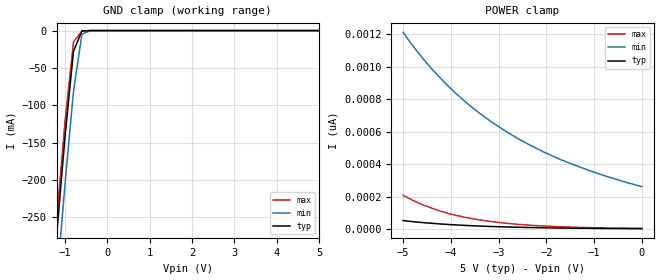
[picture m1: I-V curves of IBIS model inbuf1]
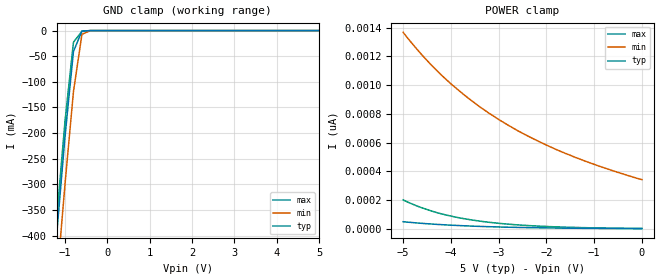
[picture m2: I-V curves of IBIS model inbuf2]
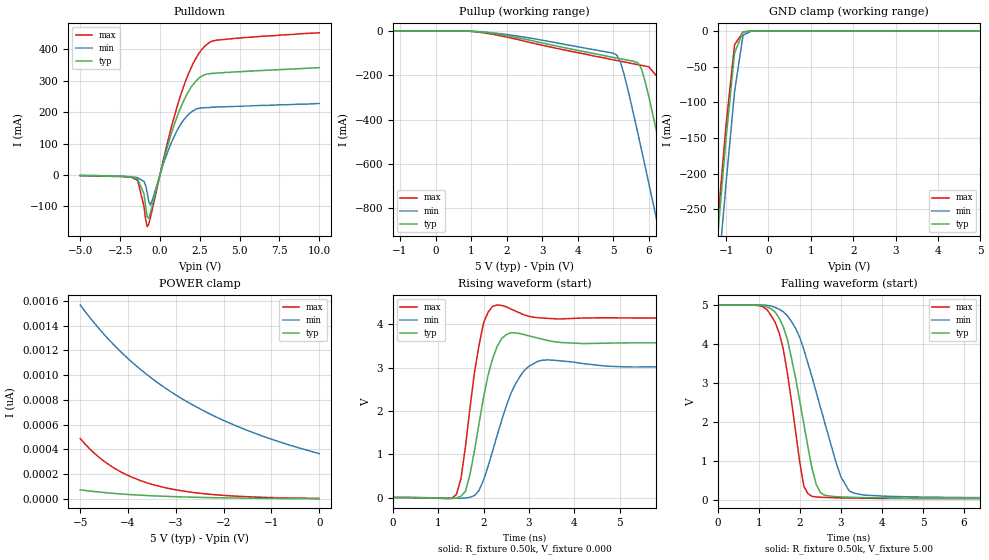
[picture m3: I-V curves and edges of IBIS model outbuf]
| IBIS file 61244l.ibs created by s2ibis2 version 1.0
| North Carolina State University Electronics Research Laboratory  1995
[IBIS ver]   2.1
[File name]   74fct16244t.ibs
[File Rev]   0.1
[Date]   Wednesday, April 16, 1997
[Source]   IDT
[Notes]   1. Temp typ=25C, min=100C, max=0C 2. Ramp rates based on 500
   ohm load
[Copyright]   Copyright 1997, Integrated Device Technology, Inc.
[Disclaimer] Integrated Device Technology, Inc. ("IDT") hereby grants the
   user of this IBIS model a non-exclusive, nontransferable
   license to use this IBIS model under the following terms.
   The user is granted this license only to use the IBIS model
   and is not granted rights to sell, copy (except as needed to
   run the IBIS model), rent, lease or sub-license the IBIS model
   in whole or in part, or in modified form to anyone.
   The User may modify the IBIS model to suit its specific
   applications, but rights to derivative works and such
   modifications shall belong to IDT.
   This IBIS model is provided on an "AS IS" basis and IDT
   makes absolutely no warranty with respect to the information
   contained herein. IDT DISCLAIMS AND CUSTOMER WAIVES ALL
   WARRANTIES, EXPRESS AND IMPLIED, INCLUDING WARRANTIES OF
   MERCHANTABILITY AND FITNESS FOR A PARTICULAR PURPOSE. THE
   ENTIRE RISK AS TO QUALITY AND PERFORMANCE IS WITH THE
   USER ACCORDINGLY, IN NO EVENT SHALL IDT BE LIABLE
   FOR ANY DIRECT OR INDIRECT DAMAGES, WHETHER IN CONTRACT OR
   TORT, INCLUDING ANY LOST PROFITS OR OTHER INCIDENTAL,
   CONSEQUENTIAL, EXEMPLARY, OR PUNITIVE DAMAGES ARISING OUT OF
   THE USE OR APPLICATION OF THE IBIS model.  Further, IDT
   reserves the right to make changes without notice to any
   product herein to improve reliability, function, or design.
   IDT does not convey any license under patent rights or
   any other intellectual property rights, including those of
   third parties. IDT is not obligated to provide maintenance
   or support for the licensed IBIS model.
|   Component IDT54/74FCT16244T/AT/CT/ET
[Component]   IDT54/74FCT16244T/AT/CT/ET
[Manufacturer]   Integrated Device Technology Inc.
[Package]
| Following package parameters are for SO48-2(TSSOP) package
|[Package]
|| variable   typ   min   max
|R_pkg   15.00m   10.00m   20.00m
|L_pkg   2.30nh   1.40nh   4.50nH
|C_pkg   0.40pF   0.35pF   0.60pF
| Following package parameters are for SO48-1(SSOP), E48-1(CERPAK) packages
| variable   typ   min   max
R_pkg   15.00m   10.00m   20.00m
L_pkg   2.90nH   1.50nH   5.60nH
C_pkg   0.40pF   0.26pF   0.50pF
[Pin]  signal_name   model_name   R_pin   L_pin   C_pin
1   1OEB   inbuf1
2   1Y1   outbuf
3   1Y2   outbuf
4   GND   GND
5   1Y3   outbuf
6   1Y4   outbuf
7   VCC   POWER
8   2Y1   outbuf
9   2Y2   outbuf
10   GND   GND
11   2Y3   outbuf
12   2Y4   outbuf
13   3Y1   outbuf
14   3Y2   outbuf
15   GND   GND
16   3Y3   outbuf
17   3Y4   outbuf
18   VCC   POWER
19   4Y1   outbuf
20   4Y2   outbuf
21   GND   GND
22   4Y3   outbuf
23   4Y4   outbuf
24   4OEB   inbuf1
25   3OEB   inbuf1
26   4A4   inbuf2
27   4A3   inbuf2
28   GND   GND
29   4A2   inbuf2
30   4A1   inbuf2
31   VCC   POWER
32   3A4   inbuf2
33   3A3   inbuf2
34   GND   GND
35   3A2   inbuf2
36   3A1   inbuf2
37   2A4   inbuf2
38   2A3   inbuf2
39   GND   GND
40   2A2   inbuf2
41   2A1   inbuf2
42   VCC   POWER
43   1A4   inbuf2
44   1A3   inbuf2
45   GND   GND
46   1A2   inbuf2
47   1A1   inbuf2
48   2OEB   inbuf1
| Models and submodels in the file (3): inbuf1 (Input), inbuf2 (Input), outbuf (3-state)
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| in   IN1   dummy_model
| oe   OE1   dummy_model
|   Model inbuf1
[Model]   inbuf1
Model_type   Input
Vinl =  0.800V
Vinh =  2.000V
C_comp   3.00pF   NA   NA
[Temperature Range]   25.00   100.00   0.000
[Voltage Range]   5.00V   4.50V   5.50V
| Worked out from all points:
|   GND clamp passes 1 mA (typ) near -0.60 V on its own axis
[GND_clamp]
| voltage   I(typ)   I(min)   I(max)
-5V       -3.018A    -3.076A    -2.999A
-1.4V     -415mA     -480mA     -394mA
-1.2V     -276mA     -341mA     -255mA
-1V       -142mA     -206mA     -122mA
-800mV    -27.87mA   -81.82mA   -15.26mA
-600mV    -480uA     -4.848mA   -551uA
-400mV    -1.016uA   -20.86uA   -873nA
5V        1.855pA    303pA      2.085pA
[POWER_clamp]
| voltage   I(typ)   I(min)   I(max)
-5V       51.46pA    1.212nA    208pA
-4.6V     39.61pA    1.056nA    150pA
-4.4V     34.75pA    987pA      128pA
-4.1V     28.53pA    894pA      99.73pA
-3.9V     25.02pA    837pA      84.6pA
-3.6V     20.53pA    760pA      66.05pA
-3.1V     14.75pA    650pA      43.65pA
-2.8V     12.09pA    593pA      34.01pA
-2.4V     9.265pA    526pA      24.35pA
-1.7V     5.808pA    428pA      13.54pA
-800mV    3.178pA    330pA      6.324pA
0V        1.855pA    261pA      3.199pA
|   Model inbuf2
[Model]   inbuf2
Model_type   Input
Vinl =  0.800V
Vinh =  2.000V
C_comp   3.00pF   NA   NA
[Temperature Range]   25.00   100.00   0.000
[Voltage Range]   5.00V   4.50V   5.50V
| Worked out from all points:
|   GND clamp passes 1 mA (typ) near -0.60 V on its own axis
[GND_clamp]
| voltage   I(typ)   I(min)   I(max)
-5V       -4.387A    -4.471A    -4.36A
-1.4V     -604mA     -698mA     -573mA
-1.2V     -402mA     -496mA     -371mA
-1V       -207mA     -300mA     -177mA
-800mV    -40.8mA    -119mA     -22.8mA
-600mV    -973uA     -7.222mA   -1.303mA
-400mV    -6.41uA    -46.07uA   -11.93uA
5V        1.965pA    393pA      2.176pA
[POWER_clamp]
| voltage   I(typ)   I(min)   I(max)
-5V       50.2pA     1.366nA    202pA
-4.6V     38.73pA    1.207nA    146pA
-4.4V     34.01pA    1.136nA    124pA
-4.1V     27.98pA    1.039nA    97.02pA
-3.6V     20.21pA    900pA      64.36pA
-3.4V     17.74pA    850pA      54.59pA
-3V       13.67pA    761pA      39.26pA
-2.6V     10.54pA    683pA      28.2pA
-2.3V     8.67pA     631pA      22pA
-1.6V     5.503pA    525pA      12.31pA
-900mV    3.5pA      437pA      6.893pA
0V        1.965pA    343pA      3.278pA
|   Model outbuf
[Model]   outbuf
Model_type   3-state
Polarity   Non-Inverting
Enable   Active-High
Vinl =  0.800V
Vinh =  2.000V
C_comp   3.00pF   NA   NA
[Temperature Range]   25.00   100.00   0.000
[Voltage Range]   5.00V   4.50V   5.50V
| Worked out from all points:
|   slope of the pulldown table from 0 to 0.75 V, typ, clamps not added: 5.47 ohm
|   slope of the pullup table from 0 to 0.75 V, typ, clamps not added: 13.5 kohm
|   GND clamp passes 1 mA (typ) near -0.59 V on its own axis
|   rising waveform, R_fixture 0.50k, V_fixture 0.000: 20-80 % time 375ps typ, 548ps min, 314ps max; typ from 0 V to 3.57 V
|   falling waveform, R_fixture 0.50k, V_fixture 5.00: 20-80 % time 538ps typ, 813ps min, 427ps max; typ from 5 V to 0.048 V
[Pulldown]
| voltage   I(typ)   I(min)   I(max)
-5V       -1mA       -1mA       -2mA
-1.4V     -12.2mA    -8mA       -16.2mA
-1V       -60mA      -20.5mA    -100mA
-800mV    -133mA     -55.02mA   -164mA
-700mV    -138mA     -84.63mA   -156mA
-600mV    -121mA     -94.98mA   -136mA
400mV     77.42mA    61.63mA    88.42mA
1.2V      202mA      153mA      238mA
2.1V      289mA      205mA      357mA
2.8V      320mA      215mA      410mA
3.6V      325mA      217mA      430mA
10V       342mA      228mA      453mA
[Pullup]
| voltage   I(typ)   I(min)   I(max)
-5V       -22.81pA   -213pA     -284pA
1V        -1.033mA   -848uA     -1.818mA
5V        -119mA     -100mA     -130mA
5.2V      -125mA     -138mA     -136mA
5.3V      -128mA     -191mA     -139mA
5.8V      -172mA     -538mA     -155mA
6V        -294mA     -685mA     -161mA
6.4V      -582mA     -982mA     -236mA
6.8V      -881mA     -1.285A    -514mA
7.2V      -1.183A    -1.591A    -812mA
7.6V      -1.487A    -1.898A    -1.114A
10V       -3.347A    -3.753A    -2.965A
[GND_clamp]
| voltage   I(typ)   I(min)   I(max)
-5V       -3.225A    -3.259A    -3.225A
-1.4V     -433mA     -494mA     -416mA
-1.2V     -289mA     -351mA     -270mA
-1V       -150mA     -213mA     -131mA
-800mV    -30.94mA   -85.08mA   -19.24mA
-600mV    -1.072mA   -5.816mA   -1.489mA
-400mV    -7.978uA   -50.35uA   -16.99uA
5V        2.361pA    421pA      2.955pA
[POWER_clamp]
| voltage   I(typ)   I(min)   I(max)
-5V       73.75pA    1.567nA    488pA
-4.8V     64.14pA    1.465nA    404pA
-4.6V     55.79pA    1.372nA    334pA
-4.4V     48.53pA    1.286nA    277pA
-4.1V     39.37pA    1.169nA    208pA
-3.6V     27.8pA     1.003nA    130pA
-3.4V     24.19pA    944pA      108pA
-3V       18.32pA    840pA      74.07pA
-2.3V     11.29pA    689pA      38.46pA
-1.7V     7.474pA    584pA      21.99pA
-900mV    4.33pA     470pA      10.5pA
0V        2.361pA    366pA      4.626pA
[Ramp]
| variable   typ   min   max
dV/dt_r   2.14/0.38n   1.81/0.55n   2.49/0.31n
dV/dt_f   2.97/0.54n   2.67/0.77n   3.27/0.44n
R_load = 0.50k
[Rising Waveform]
R_fixture = 0.50k
V_fixture = 0.000
| time   V(typ)   V(min)   V(max)
0s        0V         0V         0V
1.4ns     -14.81mV   -17.58mV   72.21mV
1.6ns     143mV      -14.15mV   1.18V
1.9ns     1.712V     165mV      3.518V
2ns       2.319V     405mV      4.035V
2.2ns     3.209V     1.076V     4.415V
2.4ns     3.672V     1.785V     4.434V
2.7ns     3.801V     2.616V     4.305V
3.2ns     3.68V      3.146V     4.151V
9.9ns     3.57V      3.022V     4.145V
[Falling Waveform]
R_fixture = 0.50k
V_fixture = 5.00
| time   V(typ)   V(min)   V(max)
0s        5V         5V         5V
1.1ns     4.986V     4.995V     4.954V
1.4ns     4.817V     4.937V     4.556V
1.7ns     4.114V     4.724V     3.248V
2.1ns     1.954V     3.857V     361mV
2.3ns     817mV      3.153V     101mV
2.5ns     203mV      2.395V     80.66mV
3ns       89.02mV    607mV      61.7mV
3.3ns     77.02mV    192mV      56.47mV
9.9ns     48.46mV    61.25mV    42.87mV
